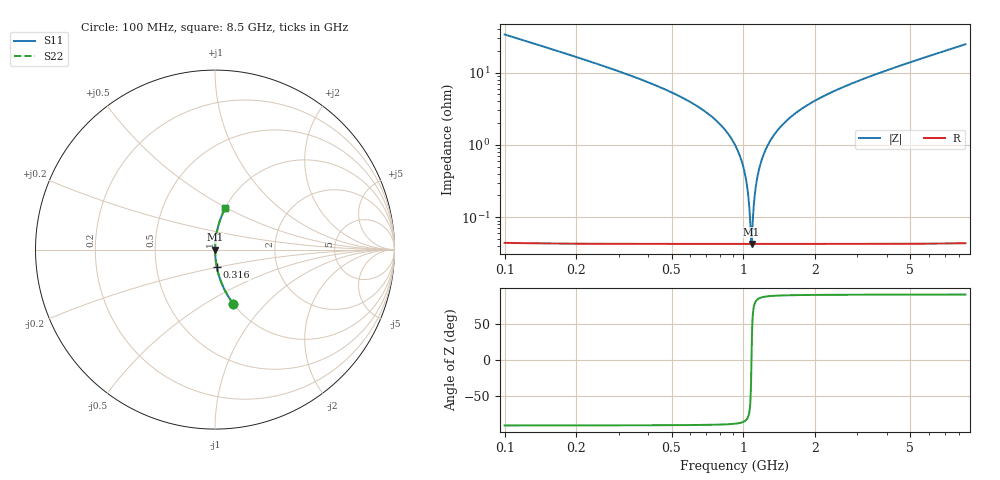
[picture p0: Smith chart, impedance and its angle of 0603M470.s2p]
! Created Wed Apr 18 16:53:06 2012
# hz S ma R 50
! 2 Port Network Data from SP1.SP block
! freq  magS11  angS11  magS21  angS21  magS12  angS12  magS22  angS22
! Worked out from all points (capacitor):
!   8401 points, 100 MHz to 8.5 GHz, reference 50 ohm
!   read as one part in series: C = 47 pF near 142 MHz
!   lowest |Z| = 42.9 mohm at 1.081 GHz (marker M1)
!   series resonance near 1.081 GHz, so ESL is about 460 pH
!   S11 on the Smith chart (normalised r, x): 100 MHz: 1.00, -0.67; 316 MHz: 1.00, -0.20; 8.5 GHz: 1.00, +0.49
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1e8  0.3181 -71.4  0.9476 18.6  0.9476 18.6  0.3181 -71.4
2.11e8  0.1525 -81.1  0.9879 8.8  0.9879 8.8  0.1525 -81.1
3.16e8  0.09749 -84.2  0.9948 5.6  0.9948 5.6  0.09749 -84.2
7.19e8  0.02623 -87.6  0.9992 1.5  0.9992 1.5  0.02623 -87.6
8.84e8  0.01268 -87.3  0.9995 0.7  0.9995 0.7  0.01268 -87.3
9.43e8  0.008574 -86.6  0.9995 0.5  0.9995 0.5  0.008574 -86.6
9.88e8  0.00564 -85.3  0.9996 0.3  0.9996 0.3  0.00564 -85.3
1.02e9  0.003647 -83.1  0.9996 0.2  0.9996 0.2  0.003647 -83.1
1.054e9  0.001623 -74.6  0.9996 0.1  0.9996 0.1  0.001623 -74.6
1.081e9  0.0004285 2.6  0.9996 -0.0  0.9996 -0.0  0.0004285 2.6
1.108e9  0.001623 74.6  0.9996 -0.1  0.9996 -0.1  0.001623 74.6
1.138e9  0.003269 82.3  0.9996 -0.2  0.9996 -0.2  0.003269 82.3
1.161e9  0.004517 84.3  0.9996 -0.3  0.9996 -0.3  0.004517 84.3
1.222e9  0.007733 86.4  0.9995 -0.4  0.9995 -0.4  0.007733 86.4
1.335e9  0.01335 87.4  0.9995 -0.8  0.9995 -0.8  0.01335 87.4
1.5e9  0.02092 87.6  0.9994 -1.2  0.9994 -1.2  0.02092 87.6
2.025e9  0.04197 87.0  0.9987 -2.4  0.9987 -2.4  0.04197 87.0
2.9e9  0.0723 85.5  0.997 -4.1  0.997 -4.1  0.0723 85.5
4.3e9  0.1163 83.1  0.9928 -6.7  0.9928 -6.7  0.1163 83.1
5.7e9  0.1582 80.7  0.987 -9.1  0.987 -9.1  0.1582 80.7
7.1e9  0.1988 78.4  0.9796 -11.5  0.9796 -11.5  0.1988 78.4
8.5e9  0.2385 76.1  0.9707 -13.8  0.9707 -13.8  0.2385 76.1
